| TEXAS INSTRUMENTS INCORPORATED
| Standard Linear and Logic Group
| IBIS Model of SN74LVC16373A
| 16-BIT TRANSPARENT D-TYPE LATCH WITH 3-STATE OUTPUTS
| This file contains package information for the following:
|  TSSOP 48-pin (DGG) package as [Component] LVC16373A_DGG
|  TVSOP 48-pin (DGV) package as [Component] LVC16373A_DGV
|  SSOP 48-pin (DL) package as [Component] LVC16373A_DL
|  VFBGA 48-pin (GQL) package as [Component] LVC16373A_GQL
|  VFBGA 48-pin (ZQL) package as [Component] LVC16373A_ZQL
| This device can be powered at the following Vccs:
|  1.8 volt Vcc
|  2.5 volt Vcc
|  2.7 volt Vcc
|  3.3 volt Vcc
| This file provides unique models under the [Model Selector] for each Vcc.
| For operation at a specific Vcc, select the appropriate model after each
| [Model Selector] keyword.
[IBIS Ver]   3.2
[Comment char]  |_char
[File Name]   sn74lvc16373a.ibs
[File Rev]   1.2 | e_die
[Date]   August 20, 2004
[Source]   Data created from TI-SPICE simulations at TI-SLL.
[Notes]   The following is an IBIS list for the LVC16373A.
   Please contact sllibis@ti.com with questions and
   comments concerning SLL IBIS models.
   This IBIS model is created from a BA (back annotated
   netlist)
   - FILE REV HISTORY
   - 1.2 ZQL package on 08/20/04
   - Power-clamp data has been deleted since there is no
   power-clamp diode in the device.
   - Due to the fact that the device is 5-V input/output
   tolerant, the pullup data has some non-monotonic warnings.
[Disclaimer] Property of Texas Instruments Incorporated.  Unauthorized
   reproduction and/or distribution is strictly prohibited.
   This product is protected under copyright law.
   Created  2003, (C) Copyright  2003, Texas Instruments
   Incorporated, All Rights Reserved
   UNLESS THERE IS A SIGNED, WRITTEN AGREEMENT TO THE
   CONTRARY, TEXAS INSTRUMENTS (TI) IS PROVIDING THE IBIS
   MODELS  AND WITHOUT ANY WARRANTY, EXPRESSED OR
   IMPLIED.  TI assumes no liability for:
   1) the accuracy of the IBIS models provided to your
   company;
   2) the proper functioning of these IBIS Models in your
   design or for any resulting applications; or
   3) infringement of patents, copyrights or intellectual
   property rights resulting from your use of these IBIS
   models.
   TI provides IBIS Models as a service to our customers.
   You and your company shall not distribute, sell or give
   these models to anyone else without prior written
   permission from TI.
   TI reserves the right to make changes to our products or
   to discontinue any semiconductor product or service
   without notice, and advises our customers to obtain the
   latest version of relevant information to verify, before
   placing orders, that the information being relied on is
   current.
   Please be aware that your receipt and use of the IBIS
   information provided shall serve as acceptance of these
   terms and conditions.  If you do not accept these terms,
   you should return or destroy the IBIS models and any
   other accompanying information immediately.
| Component LVC16373A_DGG 48-pin TSSOP
[Component]   LVC16373A_DGG
[Manufacturer]   Texas Instruments, Inc.
[Package]
|   typ   min   max
R_pkg   4.400e-02   3.800e-02   5.100e-02
L_pkg   3.019e-09   2.486e-09   4.099e-09
C_pkg   5.070e-13   3.340e-13   8.090e-13
[Pin]   signal_name   model_name   R_pin   L_pin   C_pin
1   1NOE   LVC16373A_OE   4.100e-02   4.017e-09   7.590e-13
2   1Q1   LVC16373A_OUT   4.200e-02   3.737e-09   7.920e-13
3   1Q2   LVC16373A_OUT   4.200e-02   3.480e-09   6.610e-13
4   GND   GND   3.800e-02   3.131e-09   5.750e-13
5   1Q3   LVC16373A_OUT   4.700e-02   3.122e-09   5.660e-13
6   1Q4   LVC16373A_OUT   4.300e-02   2.948e-09   5.040e-13
7   VCC   POWER   4.500e-02   2.845e-09   3.970e-13
8   1Q5   LVC16373A_OUT   4.900e-02   2.835e-09   3.940e-13
9   1Q6   LVC16373A_OUT   4.800e-02   2.715e-09   3.780e-13
10   GND   GND   5.000e-02   2.664e-09   3.630e-13
11   1Q7   LVC16373A_OUT   5.000e-02   2.585e-09   3.480e-13
12   1Q8   LVC16373A_OUT   4.900e-02   2.550e-09   3.370e-13
13   2Q1   LVC16373A_OUT   4.900e-02   2.541e-09   3.360e-13
14   2Q2   LVC16373A_OUT   5.000e-02   2.574e-09   3.480e-13
15   GND   GND   4.900e-02   2.618e-09   3.590e-13
16   2Q3   LVC16373A_OUT   4.600e-02   2.671e-09   3.750e-13
17   2Q4   LVC16373A_OUT   4.500e-02   2.754e-09   3.890e-13
18   VCC   POWER   4.400e-02   2.823e-09   4.500e-13
19   2Q5   LVC16373A_OUT   4.200e-02   2.968e-09   5.030e-13
20   2Q6   LVC16373A_OUT   5.100e-02   3.108e-09   5.350e-13
21   GND   GND   4.200e-02   3.175e-09   5.870e-13
22   2Q7   LVC16373A_OUT   4.100e-02   3.449e-09   6.780e-13
23   2Q8   LVC16373A_OUT   4.400e-02   3.766e-09   8.040e-13
24   2NOE   LVC16373A_OE   4.300e-02   4.065e-09   7.610e-13
25   2LE   LVC16373A_LE   4.100e-02   3.994e-09   7.570e-13
26   2D8   LVC16373A_IN   3.900e-02   3.649e-09   7.890e-13
27   2D7   LVC16373A_IN   3.800e-02   3.362e-09   6.600e-13
28   GND   GND   3.800e-02   3.082e-09   5.740e-13
29   2D6   LVC16373A_IN   4.400e-02   2.990e-09   5.220e-13
30   2D5   LVC16373A_IN   4.100e-02   2.917e-09   4.950e-13
31   VCC   POWER   4.300e-02   2.820e-09   4.480e-13
32   2D4   LVC16373A_IN   4.300e-02   2.699e-09   3.850e-13
33   2D3   LVC16373A_IN   4.500e-02   2.628e-09   3.720e-13
34   GND   GND   4.600e-02   2.556e-09   3.560e-13
35   2D2   LVC16373A_IN   4.600e-02   2.495e-09   3.440e-13
36   2D1   LVC16373A_IN   4.700e-02   2.487e-09   3.340e-13
37   1D8   LVC16373A_IN   4.700e-02   2.490e-09   3.350e-13
38   1D7   LVC16373A_IN   4.600e-02   2.486e-09   3.430e-13
39   GND   GND   4.500e-02   2.566e-09   3.560e-13
40   1D6   LVC16373A_IN   4.400e-02   2.639e-09   3.740e-13
41   1D5   LVC16373A_IN   4.300e-02   2.701e-09   3.860e-13
42   VCC   POWER   4.300e-02   2.817e-09   4.500e-13
43   1D4   LVC16373A_IN   4.100e-02   2.935e-09   5.010e-13
44   1D3   LVC16373A_IN   4.700e-02   3.035e-09   5.290e-13
45   GND   GND   4.300e-02   3.171e-09   5.890e-13
46   1D2   LVC16373A_IN   4.000e-02   3.415e-09   6.820e-13
47   1D1   LVC16373A_IN   4.300e-02   3.741e-09   8.090e-13
48   1LE   LVC16373A_LE   4.400e-02   4.099e-09   7.640e-13
| Component LVC16373A_DGV 48-pin TVSOP
[Component]   LVC16373A_DGV
[Manufacturer]   Texas Instruments, Inc.
[Package]
|   typ   min   max
R_pkg   7.000e-02   4.900e-02   8.500e-02
L_pkg   3.013e-09   2.743e-09   3.408e-09
C_pkg   3.710e-13   2.940e-13   5.110e-13
[Pin]   signal_name   model_name   R_pin   L_pin   C_pin
1   1NOE   LVC16373A_OE   4.900e-02   3.393e-09   4.970e-13
2   1Q1   LVC16373A_OUT   6.000e-02   3.250e-09   5.020e-13
3   1Q2   LVC16373A_OUT   7.700e-02   3.310e-09   4.510e-13
4   GND   GND   8.500e-02   3.299e-09   4.040e-13
5   1Q3   LVC16373A_OUT   8.300e-02   3.136e-09   3.600e-13
6   1Q4   LVC16373A_OUT   7.700e-02   3.019e-09   3.630e-13
7   VCC   POWER   6.500e-02   2.882e-09   3.490e-13
8   1Q5   LVC16373A_OUT   6.600e-02   2.829e-09   3.140e-13
9   1Q6   LVC16373A_OUT   6.700e-02   2.796e-09   3.140e-13
10   GND   GND   6.900e-02   2.754e-09   3.080e-13
11   1Q7   LVC16373A_OUT   7.000e-02   2.753e-09   3.010e-13
12   1Q8   LVC16373A_OUT   7.100e-02   2.745e-09   2.940e-13
13   2Q1   LVC16373A_OUT   7.000e-02   2.744e-09   2.940e-13
14   2Q2   LVC16373A_OUT   7.000e-02   2.754e-09   3.010e-13
15   GND   GND   6.900e-02   2.754e-09   3.080e-13
16   2Q3   LVC16373A_OUT   6.700e-02   2.796e-09   3.140e-13
17   2Q4   LVC16373A_OUT   6.600e-02   2.829e-09   3.140e-13
18   VCC   POWER   6.500e-02   2.883e-09   3.500e-13
19   2Q5   LVC16373A_OUT   7.500e-02   3.014e-09   3.630e-13
20   2Q6   LVC16373A_OUT   8.000e-02   3.128e-09   3.580e-13
21   GND   GND   8.400e-02   3.295e-09   4.030e-13
22   2Q7   LVC16373A_OUT   7.800e-02   3.311e-09   4.520e-13
23   2Q8   LVC16373A_OUT   6.200e-02   3.259e-09   5.010e-13
24   2NOE   LVC16373A_OE   5.200e-02   3.404e-09   4.960e-13
25   2LE   LVC16373A_LE   5.300e-02   3.397e-09   5.050e-13
26   2D8   LVC16373A_IN   6.200e-02   3.249e-09   5.110e-13
27   2D7   LVC16373A_IN   7.700e-02   3.308e-09   4.530e-13
28   GND   GND   8.200e-02   3.289e-09   4.030e-13
29   2D6   LVC16373A_IN   7.800e-02   3.121e-09   3.590e-13
30   2D5   LVC16373A_IN   7.400e-02   3.010e-09   3.630e-13
31   VCC   POWER   6.500e-02   2.883e-09   3.490e-13
32   2D4   LVC16373A_IN   6.700e-02   2.829e-09   3.140e-13
33   2D3   LVC16373A_IN   6.700e-02   2.795e-09   3.140e-13
34   GND   GND   6.900e-02   2.753e-09   3.070e-13
35   2D2   LVC16373A_IN   7.000e-02   2.753e-09   3.010e-13
36   2D1   LVC16373A_IN   7.000e-02   2.743e-09   2.940e-13
37   1D8   LVC16373A_IN   7.000e-02   2.743e-09   2.940e-13
38   1D7   LVC16373A_IN   7.000e-02   2.753e-09   3.010e-13
39   GND   GND   6.900e-02   2.754e-09   3.070e-13
40   1D6   LVC16373A_IN   6.800e-02   2.797e-09   3.140e-13
41   1D5   LVC16373A_IN   6.700e-02   2.830e-09   3.140e-13
42   VCC   POWER   6.400e-02   2.880e-09   3.490e-13
43   1D4   LVC16373A_IN   7.200e-02   3.004e-09   3.620e-13
44   1D3   LVC16373A_IN   7.800e-02   3.121e-09   3.590e-13
45   GND   GND   8.400e-02   3.296e-09   4.030e-13
46   1D2   LVC16373A_IN   7.700e-02   3.308e-09   4.510e-13
47   1D1   LVC16373A_IN   6.200e-02   3.258e-09   4.990e-13
48   1LE   LVC16373A_LE   5.300e-02   3.408e-09   4.940e-13
| Component LVC16373A_DL 48-pin SSOP
[Component]   LVC16373A_DL
[Manufacturer]   Texas Instruments, Inc.
[Package]
|   typ   min   max
R_pkg   4.800e-02   3.800e-02   5.300e-02
L_pkg   6.046e-09   5.084e-09   7.968e-09
C_pkg   8.130e-13   5.690e-13   1.157e-12
[Pin]   signal_name   model_name   R_pin   L_pin   C_pin
1   1NOE   LVC16373A_OE   4.600e-02   7.968e-09   1.017e-12
2   1Q1   LVC16373A_OUT   4.400e-02   7.299e-09   1.157e-12
3   1Q2   LVC16373A_OUT   4.300e-02   6.765e-09   1.058e-12
4   GND   GND   4.100e-02   6.269e-09   9.330e-13
5   1Q3   LVC16373A_OUT   3.800e-02   5.856e-09   8.290e-13
6   1Q4   LVC16373A_OUT   4.600e-02   5.802e-09   7.900e-13
7   VCC   POWER   5.000e-02   5.656e-09   7.380e-13
8   1Q5   LVC16373A_OUT   5.300e-02   5.500e-09   6.430e-13
9   1Q6   LVC16373A_OUT   5.200e-02   5.304e-09   6.060e-13
10   GND   GND   5.300e-02   5.189e-09   5.830e-13
11   1Q7   LVC16373A_OUT   5.100e-02   5.084e-09   5.690e-13
12   1Q8   LVC16373A_OUT   5.300e-02   5.862e-09   8.330e-13
13   2Q1   LVC16373A_OUT   5.300e-02   5.862e-09   8.330e-13
14   2Q2   LVC16373A_OUT   5.100e-02   5.084e-09   5.690e-13
15   GND   GND   5.300e-02   5.189e-09   5.830e-13
16   2Q3   LVC16373A_OUT   5.200e-02   5.304e-09   6.060e-13
17   2Q4   LVC16373A_OUT   5.300e-02   5.500e-09   6.430e-13
18   VCC   POWER   5.000e-02   5.656e-09   7.380e-13
19   2Q5   LVC16373A_OUT   4.600e-02   5.802e-09   7.900e-13
20   2Q6   LVC16373A_OUT   3.800e-02   5.856e-09   8.290e-13
21   GND   GND   4.100e-02   6.269e-09   9.330e-13
22   2Q7   LVC16373A_OUT   4.300e-02   6.765e-09   1.058e-12
23   2Q8   LVC16373A_OUT   4.400e-02   7.299e-09   1.157e-12
24   2NOE   LVC16373A_OE   4.600e-02   7.968e-09   1.017e-12
25   2LE   LVC16373A_LE   4.600e-02   7.968e-09   1.017e-12
26   2D8   LVC16373A_IN   4.400e-02   7.299e-09   1.157e-12
27   2D7   LVC16373A_IN   4.300e-02   6.765e-09   1.058e-12
28   GND   GND   4.100e-02   6.269e-09   9.330e-13
29   2D6   LVC16373A_IN   3.800e-02   5.856e-09   8.290e-13
30   2D5   LVC16373A_IN   4.600e-02   5.802e-09   7.900e-13
31   VCC   POWER   5.000e-02   5.656e-09   7.380e-13
32   2D4   LVC16373A_IN   5.300e-02   5.500e-09   6.430e-13
33   2D3   LVC16373A_IN   5.200e-02   5.304e-09   6.060e-13
34   GND   GND   5.300e-02   5.189e-09   5.830e-13
35   2D2   LVC16373A_IN   5.100e-02   5.084e-09   5.690e-13
36   2D1   LVC16373A_IN   5.300e-02   5.862e-09   8.330e-13
37   1D8   LVC16373A_IN   5.300e-02   5.862e-09   8.330e-13
38   1D7   LVC16373A_IN   5.100e-02   5.084e-09   5.690e-13
39   GND   GND   5.300e-02   5.189e-09   5.830e-13
40   1D6   LVC16373A_IN   5.200e-02   5.304e-09   6.060e-13
41   1D5   LVC16373A_IN   5.300e-02   5.500e-09   6.430e-13
42   VCC   POWER   5.000e-02   5.656e-09   7.380e-13
43   1D4   LVC16373A_IN   4.600e-02   5.802e-09   7.900e-13
44   1D3   LVC16373A_IN   3.800e-02   5.856e-09   8.290e-13
45   GND   GND   4.100e-02   6.269e-09   9.330e-13
46   1D2   LVC16373A_IN   4.300e-02   6.765e-09   1.058e-12
47   1D1   LVC16373A_IN   4.400e-02   7.299e-09   1.157e-12
48   1LE   LVC16373A_LE   4.600e-02   7.967e-09   1.017e-12
| Component LVC16373A_GQL 48-pin VFBGA
[Component]   LVC16373A_GQL
[Manufacturer]   Texas Instruments, Inc.
[Package]
|   typ   min   max
R_pkg   7.900e-02   4.500e-02   9.400e-02
L_pkg   2.264e-09   1.398e-09   2.722e-09
C_pkg   3.060e-13   1.170e-13   4.040e-13
[Pin]   signal_name   model_name   R_pin   L_pin   C_pin
A1   1NOE   LVC16373A_OE   5.100e-02   1.531e-09   2.100e-13
B2   1Q1   LVC16373A_OUT   7.300e-02   2.572e-09   3.120e-13
B1   1Q2   LVC16373A_OUT   7.100e-02   1.835e-09   2.320e-13
B3   GND   GND   9.400e-02   2.717e-09   3.830e-13
C2   1Q3   LVC16373A_OUT   8.900e-02   2.534e-09   3.500e-13
C1   1Q4   LVC16373A_OUT   7.100e-02   1.831e-09   2.310e-13
C3   VCC   POWER   9.400e-02   2.722e-09   3.920e-13
D2   1Q5   LVC16373A_OUT   9.000e-02   2.551e-09   3.520e-13
D1   1Q6   LVC16373A_OUT   7.200e-02   1.846e-09   2.440e-13
D3   GND   GND   9.400e-02   2.719e-09   4.030e-13
E2   1Q7   LVC16373A_OUT   8.900e-02   2.541e-09   3.510e-13
E1   1Q8   LVC16373A_OUT   7.200e-02   1.850e-09   2.270e-13
F1   2Q1   LVC16373A_OUT   7.200e-02   1.850e-09   2.270e-13
F2   2Q2   LVC16373A_OUT   8.900e-02   2.541e-09   3.510e-13
G3   GND   GND   9.400e-02   2.718e-09   4.040e-13
G1   2Q3   LVC16373A_OUT   7.200e-02   1.847e-09   2.440e-13
G2   2Q4   LVC16373A_OUT   9.000e-02   2.551e-09   3.520e-13
H3   VCC   POWER   9.400e-02   2.721e-09   3.920e-13
H1   2Q5   LVC16373A_OUT   7.000e-02   1.830e-09   2.310e-13
H2   2Q6   LVC16373A_OUT   8.800e-02   2.524e-09   3.500e-13
J3   GND   GND   9.300e-02   2.709e-09   3.820e-13
J1   2Q7   LVC16373A_OUT   7.100e-02   1.851e-09   2.330e-13
J2   2Q8   LVC16373A_OUT   5.600e-02   2.605e-09   3.900e-13
K1   2NOE   LVC16373A_OE   4.500e-02   1.398e-09   1.170e-13
K6   2LE   LVC16373A_IN   4.500e-02   1.512e-09   1.930e-13
J5   2D8   LVC16373A_IN   5.500e-02   2.492e-09   3.130e-13
J6   2D7   LVC16373A_IN   7.000e-02   1.821e-09   2.300e-13
J4   GND   GND   9.300e-02   2.703e-09   3.820e-13
H5   2D6   LVC16373A_IN   8.900e-02   2.529e-09   3.500e-13
H6   2D5   LVC16373A_IN   7.100e-02   1.826e-09   2.300e-13
H4   VCC   POWER   9.400e-02   2.722e-09   3.910e-13
G5   2D4   LVC16373A_IN   9.000e-02   2.551e-09   3.520e-13
G6   2D3   LVC16373A_IN   7.200e-02   1.846e-09   2.440e-13
G4   GND   GND   9.400e-02   2.719e-09   4.040e-13
F5   2D2   LVC16373A_IN   8.800e-02   2.510e-09   3.490e-13
F6   2D1   LVC16373A_IN   7.200e-02   1.850e-09   2.270e-13
E6   1D8   LVC16373A_IN   7.100e-02   1.850e-09   2.270e-13
E5   1D7   LVC16373A_IN   8.900e-02   2.529e-09   3.500e-13
D4   GND   GND   9.400e-02   2.719e-09   4.030e-13
D6   1D6   LVC16373A_IN   7.200e-02   1.847e-09   2.430e-13
D5   1D5   LVC16373A_IN   8.900e-02   2.550e-09   3.520e-13
C4   VCC   POWER   9.400e-02   2.722e-09   3.910e-13
C6   1D4   LVC16373A_IN   7.100e-02   1.827e-09   2.300e-13
C5   1D3   LVC16373A_IN   8.900e-02   2.539e-09   3.500e-13
B4   GND   GND   9.300e-02   2.705e-09   3.820e-13
B6   1D2   LVC16373A_IN   7.100e-02   1.831e-09   2.270e-13
B5   1D1   LVC16373A_IN   7.300e-02   2.685e-09   3.800e-13
A6   1LE   LVC16373A_LE   5.100e-02   1.417e-09   1.330e-13
| Component LVC16373A_ZQL 48-pin VFBGA
[Component]   LVC16373A_ZQL
[Manufacturer]   Texas Instruments, Inc.
[Package]
|   typ   min   max
R_pkg   7.900e-02   4.500e-02   9.400e-02
L_pkg   2.264e-09   1.398e-09   2.722e-09
C_pkg   3.060e-13   1.170e-13   4.040e-13
[Pin]   signal_name   model_name   R_pin   L_pin   C_pin
A1   1NOE   LVC16373A_OE   5.100e-02   1.531e-09   2.100e-13
B2   1Q1   LVC16373A_OUT   7.300e-02   2.572e-09   3.120e-13
B1   1Q2   LVC16373A_OUT   7.100e-02   1.835e-09   2.320e-13
B3   GND   GND   9.400e-02   2.717e-09   3.830e-13
C2   1Q3   LVC16373A_OUT   8.900e-02   2.534e-09   3.500e-13
C1   1Q4   LVC16373A_OUT   7.100e-02   1.831e-09   2.310e-13
C3   VCC   POWER   9.400e-02   2.722e-09   3.920e-13
D2   1Q5   LVC16373A_OUT   9.000e-02   2.551e-09   3.520e-13
D1   1Q6   LVC16373A_OUT   7.200e-02   1.846e-09   2.440e-13
D3   GND   GND   9.400e-02   2.719e-09   4.030e-13
E2   1Q7   LVC16373A_OUT   8.900e-02   2.541e-09   3.510e-13
E1   1Q8   LVC16373A_OUT   7.200e-02   1.850e-09   2.270e-13
F1   2Q1   LVC16373A_OUT   7.200e-02   1.850e-09   2.270e-13
F2   2Q2   LVC16373A_OUT   8.900e-02   2.541e-09   3.510e-13
G3   GND   GND   9.400e-02   2.718e-09   4.040e-13
G1   2Q3   LVC16373A_OUT   7.200e-02   1.847e-09   2.440e-13
G2   2Q4   LVC16373A_OUT   9.000e-02   2.551e-09   3.520e-13
H3   VCC   POWER   9.400e-02   2.721e-09   3.920e-13
H1   2Q5   LVC16373A_OUT   7.000e-02   1.830e-09   2.310e-13
H2   2Q6   LVC16373A_OUT   8.800e-02   2.524e-09   3.500e-13
J3   GND   GND   9.300e-02   2.709e-09   3.820e-13
J1   2Q7   LVC16373A_OUT   7.100e-02   1.851e-09   2.330e-13
J2   2Q8   LVC16373A_OUT   5.600e-02   2.605e-09   3.900e-13
K1   2NOE   LVC16373A_OE   4.500e-02   1.398e-09   1.170e-13
K6   2LE   LVC16373A_IN   4.500e-02   1.512e-09   1.930e-13
J5   2D8   LVC16373A_IN   5.500e-02   2.492e-09   3.130e-13
J6   2D7   LVC16373A_IN   7.000e-02   1.821e-09   2.300e-13
J4   GND   GND   9.300e-02   2.703e-09   3.820e-13
H5   2D6   LVC16373A_IN   8.900e-02   2.529e-09   3.500e-13
H6   2D5   LVC16373A_IN   7.100e-02   1.826e-09   2.300e-13
H4   VCC   POWER   9.400e-02   2.722e-09   3.910e-13
G5   2D4   LVC16373A_IN   9.000e-02   2.551e-09   3.520e-13
G6   2D3   LVC16373A_IN   7.200e-02   1.846e-09   2.440e-13
G4   GND   GND   9.400e-02   2.719e-09   4.040e-13
F5   2D2   LVC16373A_IN   8.800e-02   2.510e-09   3.490e-13
F6   2D1   LVC16373A_IN   7.200e-02   1.850e-09   2.270e-13
E6   1D8   LVC16373A_IN   7.100e-02   1.850e-09   2.270e-13
E5   1D7   LVC16373A_IN   8.900e-02   2.529e-09   3.500e-13
D4   GND   GND   9.400e-02   2.719e-09   4.030e-13
D6   1D6   LVC16373A_IN   7.200e-02   1.847e-09   2.430e-13
D5   1D5   LVC16373A_IN   8.900e-02   2.550e-09   3.520e-13
C4   VCC   POWER   9.400e-02   2.722e-09   3.910e-13
C6   1D4   LVC16373A_IN   7.100e-02   1.827e-09   2.300e-13
C5   1D3   LVC16373A_IN   8.900e-02   2.539e-09   3.500e-13
B4   GND   GND   9.300e-02   2.705e-09   3.820e-13
B6   1D2   LVC16373A_IN   7.100e-02   1.831e-09   2.270e-13
B5   1D1   LVC16373A_IN   7.300e-02   2.685e-09   3.800e-13
A6   1LE   LVC16373A_LE   5.100e-02   1.417e-09   1.330e-13
| Model LVC16373A_IN
[Model Selector]   LVC16373A_IN
LVC16373A_IN_18   1.8 volt Vcc
LVC16373A_IN_25   2.5 volt Vcc
LVC16373A_IN_27   2.7 volt Vcc
LVC16373A_IN_33   3.3 volt Vcc
| Model LVC16373A_OE
[Model Selector]   LVC16373A_OE
LVC16373A_OE_18   1.8 volt Vcc
LVC16373A_OE_25   2.5 volt Vcc
LVC16373A_OE_27   2.7 volt Vcc
LVC16373A_OE_33   3.3 volt Vcc
| Model LVC16373A_LE
[Model Selector]   LVC16373A_LE
LVC16373A_LE_18   1.8 volt Vcc
LVC16373A_LE_25   2.5 volt Vcc
LVC16373A_LE_27   2.7 volt Vcc
LVC16373A_LE_33   3.3 volt Vcc
| Model LVC16373A_OUT
[Model Selector]   LVC16373A_OUT
LVC16373A_OUT_18   1.8 volt Vcc
LVC16373A_OUT_25   2.5 volt Vcc
LVC16373A_OUT_27   2.7 volt Vcc
LVC16373A_OUT_33   3.3 volt Vcc
| Models and submodels in the file (16): LVC16373A_IN_18 (Input), LVC16373A_IN_25 (Input), LVC16373A_IN_27 (Input), LVC16373A_IN_33 (Input), LVC16373A_OE_18 (Input), LVC16373A_OE_25 (Input), LVC16373A_OE_27 (Input), LVC16373A_OE_33 (Input), LVC16373A_LE_18 (Input), LVC16373A_LE_25 (Input), LVC16373A_LE_27 (Input), LVC16373A_LE_33 (Input), LVC16373A_OUT_18 (3-state), LVC16373A_OUT_25 (3-state), LVC16373A_OUT_27 (3-state), LVC16373A_OUT_33 (3-state)
